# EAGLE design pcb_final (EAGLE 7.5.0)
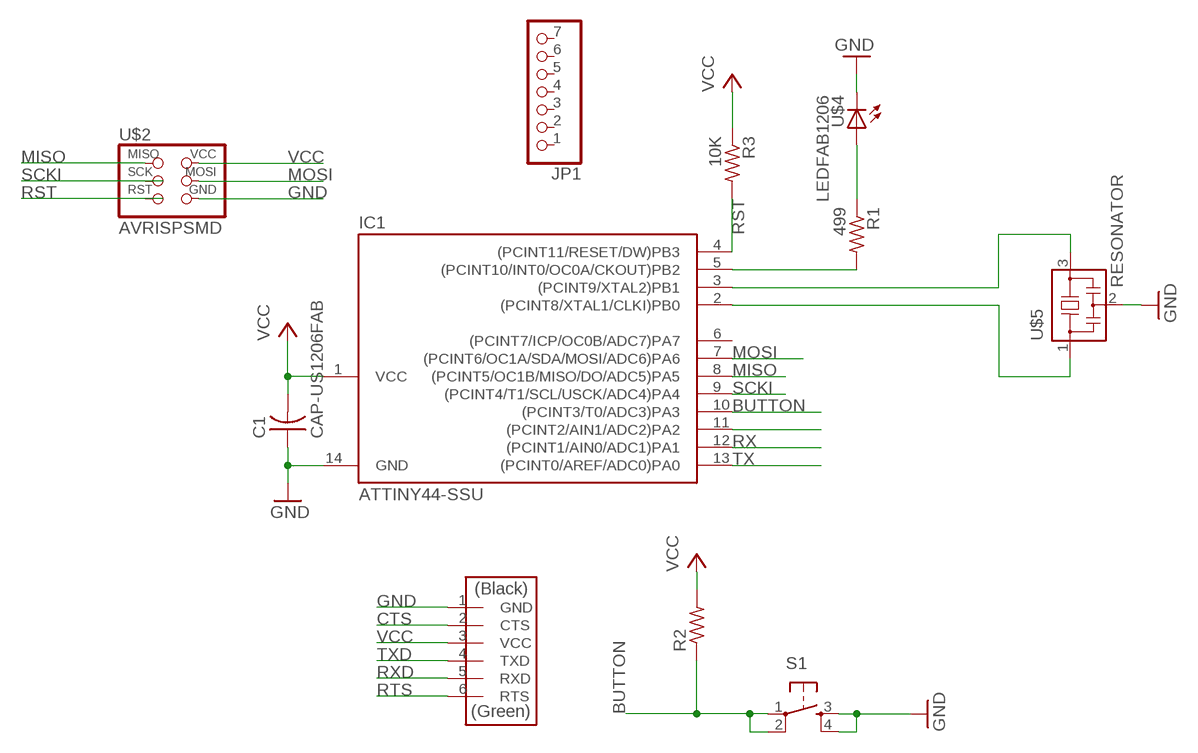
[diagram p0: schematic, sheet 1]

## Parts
C1  CAP-US1206FAB  [C1206FAB]
IC1  ATTINY44-SSU  [SOIC14]
JP1  PINHD-1X7  [1X07]
R1  499  RES-US1206  [R1206]
R2  RES-US1206FAB  [R1206FAB]
R3  10K  RES-US1206FAB  [R1206FAB]
S1  6MM_SWITCH6MM_SWITCH  [6MM_SWITCH]
U$2  AVRISPSMD  [2X03SMD]
U$3  FTDI-SMD-HEADER  [1X06SMD]
U$4  LEDFAB1206  [LED1206FAB]
U$5  RESONATOR  [EFOBM]

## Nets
BUTTON: IC1.10((PCINT3/T0/ADC3)PA3) R2.1 S1.1(P) S1.2(P1)
CTS: U$3.2(CTS)
GND: C1.1 IC1.14(GND) S1.3(S) S1.4(S1) U$2.6(GND) U$3.1(GND) U$4.2(C) U$5.2
MISO: IC1.8((PCINT5/OC1B/MISO/DO/ADC5)PA5) U$2.1(MISO)
MOSI: IC1.7((PCINT6/OC1A/SDA/MOSI/ADC6)PA6) U$2.4(MOSI)
N$1: IC1.3((PCINT9/XTAL2)PB1) U$5.3
N$2: IC1.2((PCINT8/XTAL1/CLKI)PB0) U$5.1
N$3: IC1.5((PCINT10/INT0/OC0A/CKOUT)PB2) R1.2
N$4: IC1.11((PCINT2/AIN1/ADC2)PA2)
N$5: R1.1 U$4.1(A)
RST: IC1.4((PCINT11/RESET/DW)PB3) R3.2
RTS: U$3.6(RTS)
RX: IC1.12((PCINT1/AIN0/ADC1)PA1)
RXD: U$3.5(RXD)
SCKI: IC1.9((PCINT4/T1/SCL/USCK/ADC4)PA4)
TX: IC1.13((PCINT0/AREF/ADC0)PA0)
TXD: U$3.4(TXD)
VCC: C1.2 IC1.1(VCC) R2.2 R3.1 U$2.2(VCC) U$3.3(VCC)
Unconnected: IC1.6((PCINT7/ICP/OC0B/ADC7)PA7) JP1.1 JP1.2 JP1.3 JP1.4 JP1.5 JP1.6 JP1.7 U$2.3(SCK) U$2.5(RST)

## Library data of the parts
C1 = fab:CAP-US
IC1 = fab:ATTINY44
JP1 = pinhead:PINHD-1X7: PIN HEADER
R1-R3 = fab:RES-US: Resistor (US Symbol)
S1 = fab:6MM_SWITCH: OMRON SWITCH
U$2 = fab:AVRISP
U$3 = fab:FTDI-SMD-HEADER
U$4 = fab:LED: LED
U$5 = fab:RESONATOR

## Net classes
0 default: clearance 0.205 mm

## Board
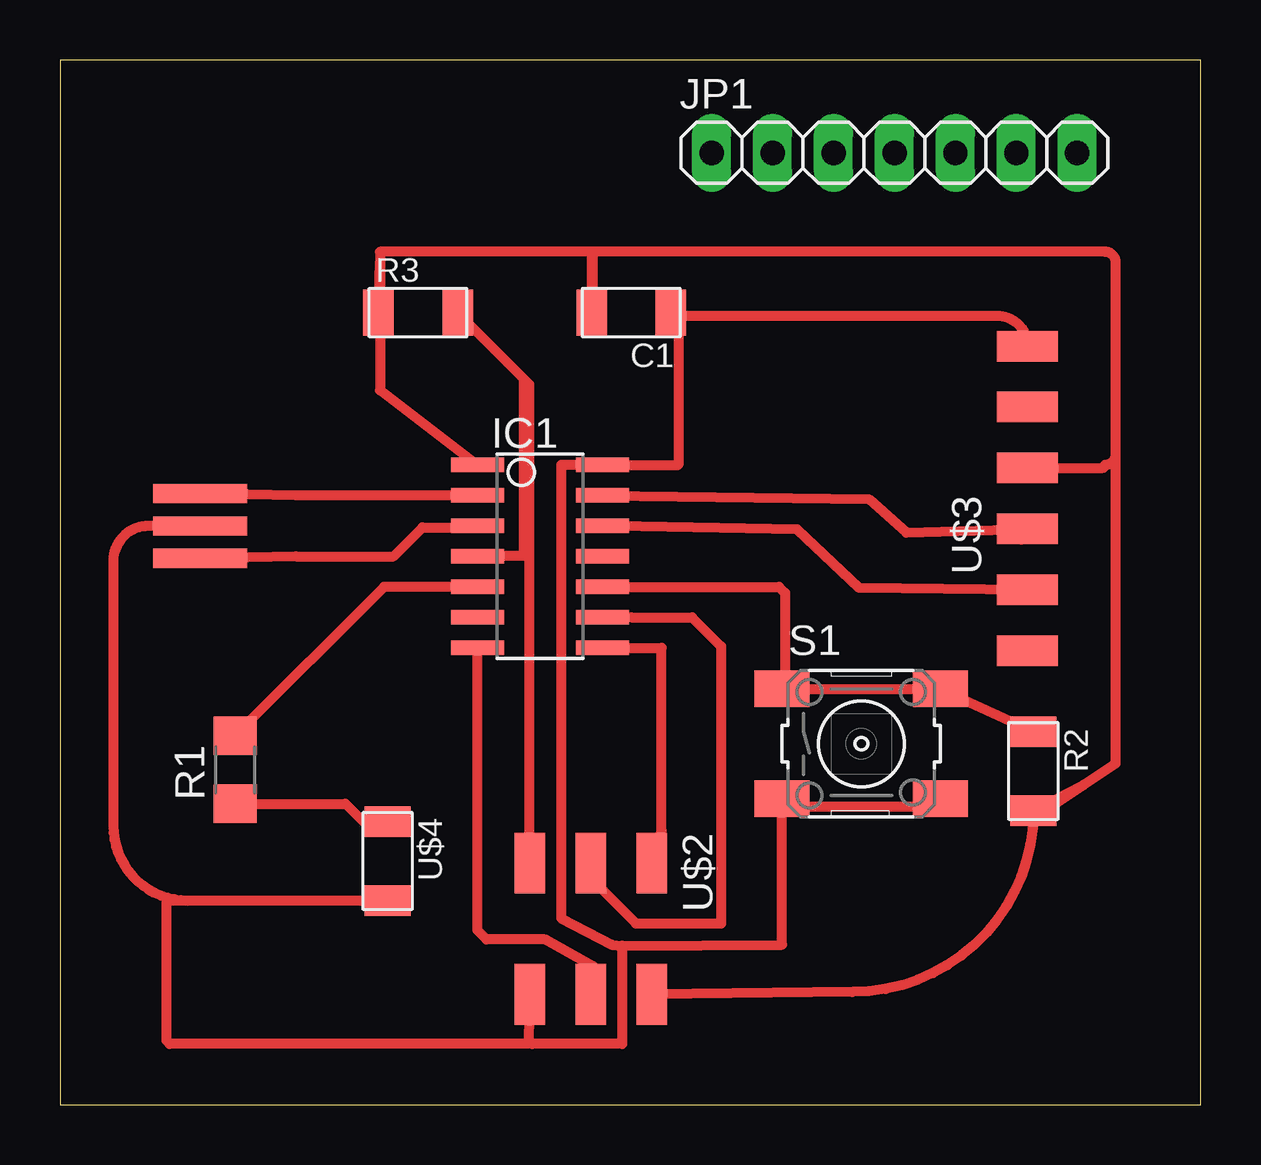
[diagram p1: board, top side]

Size 47.55 x 43.55 mm. Coordinates in mm from the lower left corner, seen from the top.
Outline: 0,0 47.55,0 47.55,43.55 0,43.55 0,0
Copper layers (1*16): Top 0.035mm / dielectric 1.5mm / Bottom 0.035mm
Design rules "SparkFun *": minimum track width 8mil, minimum drill 20mil, track to track 16mil, track to pad 16mil, pad to pad 16mil, via to via 16mil, smd to smd 16mil, copper to edge 8mil, drill to drill 8mil, minimum pad ring 12mil, minimum via ring 10mil, stop-mask expansion 4mil, vias tented up to drill 20mil, thermal gap 10mil

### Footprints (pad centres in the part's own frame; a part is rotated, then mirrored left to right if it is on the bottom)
C1206FAB = smd 1.27 x 1.905: 1 -1.651,0; 2 1.651,0
SOIC14 = smd 0.61 x 2.21: 1 -3.81,-2.603; 2 -2.54,-2.603; 3 -1.27,-2.603; 4 0,-2.603; 5 1.27,-2.603; 6 2.54,-2.603; 7 3.81,-2.603; 8 3.81,2.603; 9 2.54,2.603; 10 1.27,2.603; 11 0,2.603; 12 -1.27,2.603; 13 -2.54,2.603; 14 -3.81,2.603
1X07 = drill 1.016 long: 1 -7.62,0; 2 -5.08,0; 3 -2.54,0; 4 0,0; 5 2.54,0; 6 5.08,0; 7 7.62,0
R1206 = smd 1.6 x 1.803: 1 -1.422,0; 2 1.422,0
R1206FAB = smd 1.27 x 1.905: 1 -1.651,0; 2 1.651,0
6MM_SWITCH = smd 2.286 x 1.524: 1 -3.302,2.286; 2 3.302,2.286; 3 -3.302,-2.286; 4 3.302,-2.286
2X03SMD = smd 2.54 x 1.27: 1 -2.54,2.54; 2 2.92,2.54; 3 -2.54,0; 4 2.92,0; 5 -2.54,-2.54; 6 2.92,-2.54
1X06SMD = smd 2.54 x 1.27: 1 0,6.35; 2 0,3.81; 3 0,1.27; 4 0,-1.27; 5 0,-3.81; 6 0,-6.35
LED1206FAB = smd 1.27 x 1.905: 1 -1.651,0; 2 1.651,0
EFOBM = smd 0.8 x 3.9: 1 -1.35,0; 2 0,0; 3 1.35,0

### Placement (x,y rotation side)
C1  23.81,33.02 180 top
IC1  20,22.86 270 top
JP1  34.78,39.68 0 top
R1  7.3,13.97 90 top
R2  40.58,13.91 270 top
R3  14.92,33.02 0 top
S1  33.4,15.05 0 top
U$2  22.13,7.53 270 top
U$3  40.32,25.27 0 top
U$4  13.65,10.16 270 top
U$5  5.84,24.13 270 top

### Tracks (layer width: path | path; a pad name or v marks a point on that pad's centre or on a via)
BUTTON
  Top 0.406: IC1.10 29.97,21.59 30.23,21.34 30.23,17.46 S1.1 | S1.1 30.67,17.34 | S1.1 S1.2 R2.1
GND
  Top 0.406: 19.68,2.54 23.43,2.54 23.43,6.63 | 19.68,2.54 19.56,2.67 U$2.6 | 19.68,2.54 4.57,2.54 4.45,2.67 4.45,8.45 4.51,8.51 5.33,8.51 | U$4.2 5.33,8.51 | C1.1 25.78,32.7 | 25.78,32.7 25.78,26.67 IC1.14 20.89,26.67 20.89,7.78 23,6.67 23.43,6.63 | 25.78,32.7 25.97,32.89 39.05,32.89 arc-90 U$3.1 | U$5.2 3.68,24.13 arc90 2.22,22.67 2.22,11.62 arc90 5.33,8.51 | 23.43,6.63 30.1,6.67 S1.3 30.23,12.45 36.7,12.45 S1.4
MISO
  Top 0.406: U$2.1 25.08,11.43 25.08,19.05 IC1.8
MOSI
  Top 0.406: U$2.4 22.23,4.83 22.23,5.78 20.23,6.89 17.78,6.89 17.4,7.27 IC1.7
N$1
  Top 0.406: U$5.3 9.84,22.86 13.9,22.86 15.11,24.07 17.34,24.07 IC1.3
N$2
  Top 0.406: IC1.2 9.84,25.4 U$5.1
N$3
  Top 0.406: IC1.5 13.5,21.59 R1.2
N$5
  Top 0.406: R1.1 11.9,12.55 12.89,11.56 13.4,11.56 U$4.1
N$9
  Top 0.406: 22.51,10.1 22.54,9.02 24,7.56 27.56,7.56 27.56,19.11 26.35,20.32 23.81,20.32
RST
  Top 0.406: IC1.4 17.43,22.89 19.34,22.89 19.34,30.26 R3.2 19.56,30.04 19.56,10.22
RXD
  Top 0.406: U$3.5 33.31,21.55 30.74,23.98 23.14,24.12
TXD
  Top 0.406: 40.07,23.56 U$3.4 35.27,23.85 33.72,25.25 22.54,25.4
VCC
  Top 0.406: U$2.2 33.02,4.7 arc90 R2.2 42.67,13.34 | 44.01,27.11 arc-90 43.56,26.67 arc-90 43.43,26.54 U$3.3 | 44.01,27.11 44.01,35.12 arc90 43.56,35.56 22.23,35.56 | 22.23,35.56 arc90 22.16,35.5 C1.2 arc90 22.23,33.08 22.23,35.56 | 22.23,35.56 13.34,35.56 13.34,35.12 | 13.34,35.12 13.34,29.78 IC1.1 17.34,26.67 | 42.67,13.34 44.01,14.22 44.01,27.11 | 42.67,13.34 41.34,12.45 | R3.1 13.34,35.12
